//FC655.AWL
// ***************************************************************************

FUNCTION "FC_SR_JOB_USER" : VOID
TITLE = Querkopplung Call-Schnittstelle f. Anwender

AUTHOR: 	SIEMENS
FAMILY: 	SISTARS7
VERSION: 	4.02

//KNOW_HOW_PROTECT

// Datum	 Name			Aktion
// ---------------------------------------------------------------------------
// 19.06.99 Mahler		Neu
//
// Return: 		VKE0		OK
//			VKE1		Fehler
//			iRetVal	>0	OK: Wert=bearbeiteter Job
//		   			<0	Fehler	-1	Keinen freien Job mit iPCU==0 gefunden
//								-2	"XC_JOB" hat keine Datensätze
//								-3	iMode falsch
//								-4	PCU nicht in "XC_PCU" enthalten oder <1 oder >200

VAR_INPUT

	iMode			: INT;				//1: Set Job Data
									//2: Set ActTime to zero

	iJob			: INT;				//1..32:	System-Job fuer FC
									//33..64:   System-Job fuer Software
									//65..DB705.iActSum: User Job 1..256
									//=0: every job 1 .. 32
									//<0: every job 65 ...
	iPCU			: INT;				//1..200

	iType			: INT;				//Job-Type
									//50=DB-Send, 51=DX-Send
									//66=Send_Time S5, 68=Send_Time S7
									//52=DB-Fetch, 53=DX-Fetch

	boEnable		: BOOL;				//1: Enable Job, Disable Job
	boTmpJob		: BOOL;				//temp. Job

	iSrc_DType		: INT;				//Source Data Type, 2=byte, 4=word,...
	iSrc_AREA		: INT;            		//Source 0x80..0x84 = P,E,A,M,DB
	iSrc_DB		: INT;				//Source D/P/I/O/F-Number
	dSrcByte		: DINT;				//Source Byte Address
	iSrcBit		: INT;				//Source Bit Address
	iSrc_Num		: INT;				//Number of Data Type 1..400

	iDest_DType		: INT;				//Destination Data Type, 2=byte, 4=word,...
	iDest_AREA		: INT;            		//Destination 0x80..0x84 = P,E,A,M,DB
	iDest_DB		: INT;				//Destination D/P/I/O/F-Number
	dDestByte		: DINT;				//Destination Byte Address
	iDestBit		: INT;				//Destination Bit Address

	iTime			: INT		:= 10;		//Sollzeit (s)
	iActTime		: INT		:= 10;		//Sollzeit (s)

	boTms			: BOOL;				//1: TimeBase 100 ms
	boTsec		: BOOL;				//1: TimeBase sec
	boTmin		: BOOL;				//1: TimeBase min
END_VAR

VAR_OUTPUT
	iRetVal		: INT;				//>0: handled Job, <0: ErrorCode
									//-1: No free job found
									//-2:	 no jobs in "XC_JOB"

END_VAR

VAR_TEMP
	dwAR1			: DWORD;
	i			: INT;
	iend			: INT;
END_VAR

BEGIN


NETWORK
TITLE = AR1 retten
// ===========================================================================

	TAR1	#dwAR1;

NETWORK
TITLE = Job prüfen
// ===========================================================================

	L	"XC_JOB_SR".iActSum;
	L	0;
	<=I;
	SPB	ER02;

	L	#iJob;
	L	0;
	<=I;
	SPB	JOBE;

	L	#iJob;
	L	"XC_JOB_SR".iActSum;
	<=I;
	SPB	JOBE;

JOB0:	L	0;
	T	#iJob;



JOBE:	NOP	0;


NETWORK
TITLE = Zeiger auf stellen, bei Job=0 Job suchen
// ===========================================================================
	L	#iMode;
	L	2;
	<>I;
	SPB	M1S;
      L     #iJob;			   //Job muss eingetragen sein bei MODE=2
      L 	0;
      ==I;
	spb   ER03;

M1S:	L	#iJob;	                //Job-Nummer vorgegeben 1 ... 320
	L	0;
	>I;
	SPB	JSAR;
      L     #iJob;			   //Job suchen von 1 .. 32
      L 	0;
      ==I;
	spb   JS0;
      L     #iJob;			   //Job suchen von 65 .. 320
      L 	0;
      <I;
	spb   JS1;

JS0:	L	"XC_JOB_SR".iOffsetSys;
	SLD	3;
	LAR1;						//Zeiger auf ersten Datensatz

	L	1;
      T     #iJob;
	L	"XC_JOB_SR".iSys;
	SRW   1;
	T     #iend;
      spb   JSLP;

JS1:	L	"XC_JOB_SR".iOffset;
	SLD	3;
	LAR1;						//Zeiger auf ersten Datensatz

	L	"XC_JOB_SR".iSys;
	+	1;
      T     #iJob;
	L	"XC_JOB_SR".iActSum;
	T     #iend;

JSLP:	L	#iJob;
	L	#iend;
	>I;
	SPB	ER01;					//Keinen Job gefunden

	L	DBW	[AR1, P#0.0];		//#iPCU
	L	0;
	==I;
	SPB	JSE;

	L	"XC_JOB_SR".iLen;
	SLW	3;
	+AR1;

	L	#iJob;
	+	1;
      T     #iJob;
	SPA	JSLP;

JSAR:	L	#iJob;
	+	-1;
	L	"XC_JOB_SR".iLen;
	*D;
	L	"XC_JOB_SR".iOffsetSys;
	+D;
	SLD	3;
	LAR1;

JSE:	NOP	0;


NETWORK
TITLE = Mode = 1: Job-Daten setzen
// ===========================================================================

	L	#iMode;
	L	1;
	<>I;
	SPB	M1E;

	L	#iPCU;
	T	DBW	[AR1, P#0.0];

	L	#iType;
	T	DBB	[AR1, P#2.0];

	U	#boEnable;
	=	DBX	[AR1, P#3.0];

	U	#boTmpJob;
	=	DBX	[AR1, P#3.7];

	U	#boTms;
	UN	#boTsec;
	=	DBX	[AR1, P#3.4];
	U	#boTmin;
	UN	#boTsec;
	=	DBX	[AR1, P#3.5];

	L	#iSrc_DType;
	T	DBB	[AR1, P#4.0];

	L	#iSrc_AREA;
	T	DBB	[AR1, P#5.0];

	L	#iSrc_DB;
	T	DBW	[AR1, P#6.0];

	L	#dSrcByte;
	T	DBD	[AR1, P#8.0];

	L	#iSrcBit;
	T	DBB	[AR1, P#12.0];

	L	#iSrc_Num;
	T	DBW	[AR1, P#14.0];

	L	#iDest_DType;
	T	DBB	[AR1, P#16.0];

	L	#iDest_AREA;
	T	DBB	[AR1, P#17.0];

	L	#iDest_DB;
	T	DBW	[AR1, P#18.0];

	L	#dDestByte;
	T	DBD	[AR1, P#20.0];

	L	#iDestBit;
	T	DBB	[AR1, P#24.0];

	L	#iTime;
	T	DBW	[AR1, P#28.0];

	L	#iActTime;
	T	DBW	[AR1, P#30.0];

	SPA	OK;

M1E:	NOP	0;


NETWORK
TITLE = Mode = 2: Zeit auf 0 setzen
// ===========================================================================

	L	#iMode;
	L	2;
	<>I;
	SPB	M2E;

	L	#iActTime;
	T	DBW	[AR1, P#30.0];			//#iActTime;

	SPA	OK;

M2E:	NOP	0;


NETWORK
TITLE = OK/Errors
// ===========================================================================
	L	-3;					//Mode falsch
	SPA	RVAL;

ER01:	L	-1;					//Keinen freien Job gefunden
	SPA	RVAL;

ER02:	L	-2;					//Keine Jobs in "XC_JOB"
	SPA	RVAL;

ER03:	L     -3;					//Falsche Parameter
	SPA	RVAL;

ER04:	L	-4;					//PCU falsch
	SPA	RVAL;

OK:	L	#iJob;
RVAL:	T	#iRetVal;


NETWORK
TITLE = AR1 zurück, ENDE
// ===========================================================================

	LAR1	#dwAR1;

	L	#iRetVal;
	L	0;
	<I;					//VKE

END_FUNCTION

